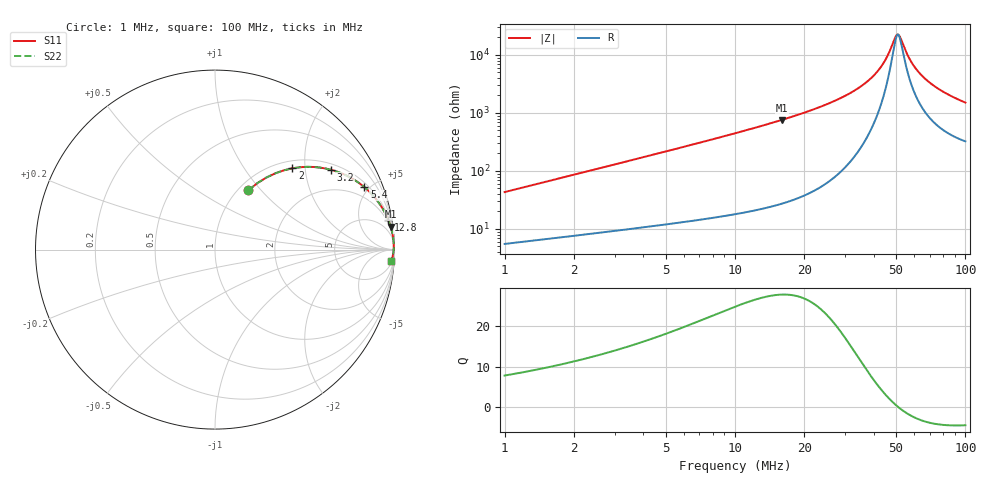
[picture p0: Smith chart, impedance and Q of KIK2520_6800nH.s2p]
!version-2
!date-01.2022
!Series
# MHz S RI R 50
!Freq ReS11 ImS11 ReS21 ImS21 ReS12 ImS12 ReS22 ImS22
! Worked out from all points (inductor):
!   496 points, 1 MHz to 100 MHz, reference 50 ohm
!   read as one part in series: L = 6.8 uH near 1.4 MHz
!   highest Q = 27.8 at 16 MHz (marker M1), where L = 7.54 uH
!   self-resonance near 51 MHz
!   S11 on the Smith chart (normalised r, x): 1 MHz: 1.11, +0.85; 2 MHz: 1.15, +1.71; 3.2 MHz: 1.19, +2.75; 5.4 MHz: 1.25, +4.67; 12.8 MHz: 1, +12; 100 MHz: 7, -29
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1  0.1858 0.3299  0.8142 -0.3299  0.8142 -0.3299  0.1858 0.3299
2  0.4307 0.4528  0.5693 -0.4528  0.5693 -0.4528  0.4307 0.4528
3.2  0.6448 0.4452  0.3552 -0.4452  0.3552 -0.4452  0.6448 0.4452
4.2  0.7532 0.402  0.2468 -0.402  0.2468 -0.402  0.7532 0.402
5.4  0.8324 0.3478  0.1676 -0.3478  0.1676 -0.3478  0.8324 0.3478
8.2  0.9189 0.252  0.0811 -0.252  0.0811 -0.252  0.9189 0.252
12.8  0.9658 0.1642  0.0342 -0.1642  0.0342 -0.1642  0.9658 0.1642
16  0.9785 0.1282  0.0215 -0.1282  0.0215 -0.1282  0.9785 0.1282
17.6  0.9825 0.1144  0.0175 -0.1144  0.0175 -0.1144  0.9825 0.1144
34  0.9955 0.0379  0.00447 -0.0379  0.00447 -0.0379  0.9955 0.0379
39  0.9961 0.0247  0.00389 -0.0247  0.00389 -0.0247  0.9961 0.0247
43  0.9962 0.0156  0.00383 -0.0156  0.00383 -0.0156  0.9962 0.0156
46  0.996 0.00939  0.00396 -0.00939  0.00396 -0.00939  0.996 0.00939
49.6  0.9957 0.00255  0.00427 -0.00255  0.00427 -0.00255  0.9957 0.00255
50.6  0.9956 0.000745  0.00438 -0.000745  0.00438 -0.000745  0.9956 0.000745
52  0.9954 -0.00172  0.00455 0.00172  0.00455 0.00172  0.9954 -0.00172
55.6  0.9949 -0.00776  0.00508 0.00776  0.00508 0.00776  0.9949 -0.00776
58.8  0.9944 -0.0128  0.00564 0.0128  0.00564 0.0128  0.9944 -0.0128
67  0.9926 -0.0247  0.00742 0.0247  0.00742 0.0247  0.9926 -0.0247
74.4  0.9906 -0.0343  0.00936 0.0343  0.00936 0.0343  0.9906 -0.0343
83.6  0.9878 -0.0453  0.0122 0.0453  0.0122 0.0453  0.9878 -0.0453
100  0.9819 -0.0628  0.0181 0.0628  0.0181 0.0628  0.9819 -0.0628
